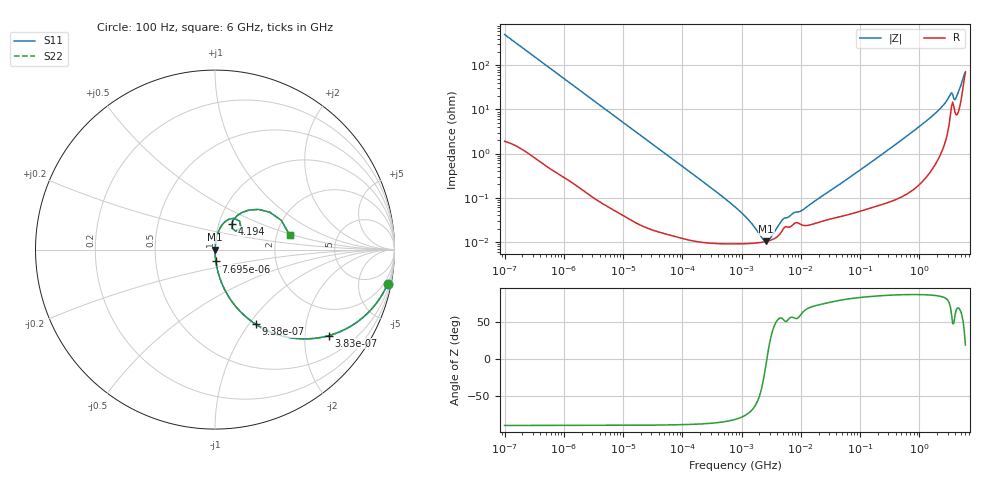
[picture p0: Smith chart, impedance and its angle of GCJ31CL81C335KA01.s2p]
!Murata Part Number: GCJ31CL81C335KA01
!These Parameters are Measured in Series Mode Connection
!Data Generated on Mar 13, 2026
!  o--ll--o
!Port1  Port2
!  o------o
!Operation Temp=25[degC], DC Bias Voltage=0[V]
!Freq. Start=100[Hz] Stop=6[GHz] 401[Steps]
# Hz S RI R 50
!Freq.(Hz) S11(Real) S11(Imag) S21(Real) S21(Imag) S12(Real) S12(Imag) S22(Real) S22(Imag)
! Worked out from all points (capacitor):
!   401 points, 100 Hz to 6 GHz, reference 50 ohm
!   read as one part in series: C = 3.16 uF near 109 Hz
!   lowest |Z| = 10.2 mohm at 2.595 MHz (marker M1)
!   series resonance near 2.672 MHz, so ESL is about 1.1 nH
!   S11 on the Smith chart (normalised r, x): 100 Hz: 1, -10; 383 Hz: 1.01, -2.63; 938 Hz: 1.01, -1.08; 7.695 kHz: 1.00, -0.13; 4.194 GHz: 1.15, +0.34; 6 GHz: 2.36, +0.47
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100  0.9612 -0.1912  0.0388 0.1912  0.0388 0.1912  0.9612 -0.1912
205  0.857 -0.3476  0.143 0.3476  0.143 0.3476  0.857 -0.3476
383  0.6338 -0.4792  0.3662 0.4792  0.3662 0.4792  0.6338 -0.4792
600  0.4159 -0.4902  0.5841 0.4902  0.5841 0.4902  0.4159 -0.4902
938  0.2268 -0.4159  0.7732 0.4159  0.7732 0.4159  0.2268 -0.4159
2008  0.0613 -0.2369  0.9387 0.2369  0.9387 0.2369  0.0613 -0.2369
7695  0.00485 -0.0659  0.9951 0.0659  0.9951 0.0659  0.00485 -0.0659
40335  0.000328 -0.0127  0.9997 0.0127  0.9997 0.0127  0.000328 -0.0127
774597  8.99e-05 -0.000613  0.9999 0.000613  0.9999 0.000613  8.99e-05 -0.000613
1267578  9.11e-05 -0.000318  0.9999 0.000318  0.9999 0.000318  9.11e-05 -0.000318
2268635  9.82e-05 -6.44e-05  0.9999 6.44e-05  0.9999 6.44e-05  9.82e-05 -6.44e-05
2594782  0.000102 -1.15e-05  0.9999 1.15e-05  0.9999 1.15e-05  0.000102 -1.15e-05
3103719  0.000109 5.98e-05  0.9999 -5.98e-05  0.9999 -5.98e-05  0.000109 5.98e-05
5079039  0.000198 0.000267  0.9998 -0.000267  0.9998 -0.000267  0.000198 0.000267
1.039699e7  0.000242 0.000451  0.9998 -0.000451  0.9998 -0.000451  0.000242 0.000451
1.555665e7  0.00025 0.00072  0.9998 -0.00072  0.9998 -0.00072  0.00025 0.00072
3.124326e8  0.000956 0.0127  0.999 -0.0127  0.999 -0.0127  0.000956 0.0127
1.637704e9  0.00915 0.0693  0.9908 -0.0693  0.9908 -0.0693  0.00915 0.0693
3.205649e9  0.0766 0.1686  0.9234 -0.1686  0.9234 -0.1686  0.0766 0.1686
4.193612e9  0.0927 0.1444  0.9073 -0.1444  0.9073 -0.1444  0.0927 0.1444
5.016141e9  0.1916 0.2208  0.8084 -0.2208  0.8084 -0.2208  0.1916 0.2208
6e9  0.4156 0.082  0.5844 -0.082  0.5844 -0.082  0.4156 0.082
